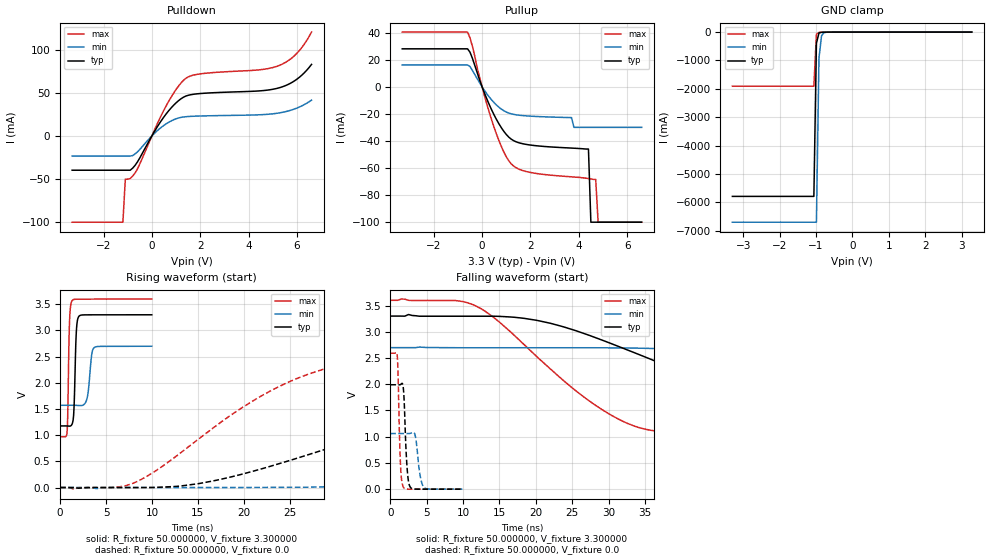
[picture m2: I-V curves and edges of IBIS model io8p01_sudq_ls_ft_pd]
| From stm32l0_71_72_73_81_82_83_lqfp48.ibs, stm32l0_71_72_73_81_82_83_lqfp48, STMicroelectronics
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|   Model io8p01_sudq_ls_ft_pd
[Model]  io8p01_sudq_ls_ft_pd
Model_type I/O
Polarity   Non-Inverting
Enable   Active-Low
Vinl =   0.990000V
Vinh =   2.310000V
Vmeas =  1.650000V
Cref =   50.000000pF
Rref =   100.000000M
Vref =   0.0V
C_comp   2.343000pF   2.309800pF   2.393900pF
[Temperature Range]   25.000000   0.125000k   -40.000000
[Pullup Reference]   3.300000V   2.700000V   3.600000V
[Pulldown Reference]   0.0V   0.0V   0.0V
[POWER Clamp Reference]   3.300000V   2.700000V   3.600000V
[GND Clamp Reference]   0.0V   0.0V   0.0V
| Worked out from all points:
|   slope of the pulldown table from 0 to 0.495 V, typ, clamps not added: 22.6 ohm
|   slope of the pullup table from 0 to 0.495 V, typ, clamps not added: 23.9 ohm
|   GND clamp passes 1 mA (typ) near -0.64 V on its own axis
|   rising waveform, R_fixture 50.000000, V_fixture 3.300000: 20-80 % time 207ps typ, 362ps min, 164ps max; typ from 1.18 V to 3.3 V
|   rising waveform, R_fixture 50.000000, V_fixture 0.0: 20-80 % time 27.1ns typ, 59.7ns min, 13.6ns max; typ from 0 V to 1.99 V
|   falling waveform, R_fixture 50.000000, V_fixture 3.300000: 20-80 % time 24.5ns typ, 54ns min, 13.4ns max; typ from 3.3 V to 1.18 V
|   falling waveform, R_fixture 50.000000, V_fixture 0.0: 20-80 % time 380ps typ, 551ps min, 301ps max; typ from 1.99 V to 0 V
[Pulldown]
|Voltage   I(typ)   I(min)   I(max)
-3.3V     -39.8mA    -23.38mA   -100mA
-1.2V     -39.8mA    -23.38mA   -100mA
-1.1V     -39.8mA    -23.38mA   -50.11mA
-900mV    -39.8mA    -23.38mA   -49.43mA
-700mV    -34.25mA   -21mA      -43.13mA
600mV     25.84mA    14.18mA    35.34mA
1V        38.32mA    19.82mA    53.81mA
1.4V      46.09mA    22.19mA    66.63mA
2V        49.05mA    23.02mA    71.83mA
5.2V      55.23mA    26.32mA    80.92mA
6V        65.76mA    32.26mA    95.84mA
6.6V      82.81mA    41.44mA    120.2mA
[Pullup]
|Voltage   I(typ)   I(min)   I(max)
-3.3V     27.97mA    16.07mA    40.33mA
-600mV    27.97mA    16.07mA    40.33mA
400mV     -17.21mA   -9.813mA   -24.69mA
800mV     -30.32mA   -16.54mA   -44.19mA
1.2V      -38.62mA   -19.99mA   -56.79mA
3.7V      -45.29mA   -22.8mA    -66.51mA
3.8V      -45.39mA   -30mA      -66.64mA
4.4V      -46mA      -30mA      -67.77mA
4.5V      -100mA     -30mA      -68.06mA
4.7V      -100mA     -30mA      -68.41mA
4.8V      -100mA     -30mA      -100mA
6.6V      -100mA     -30mA      -100mA
[GND_clamp]
|Voltage   I(typ)   I(min)   I(max)
-3.3V     -5.787A    -6.696A    -1.906A
-1.06V    -5.787A    -6.696A    -1.906A
-990mV    -393.4mA   -6.696A    -70.76mA
-920mV    -33.04mA   -919.4mA   -10.91mA
-850mV    -6.842mA   -131.3mA   -6.529mA
-780mV    -3.49mA    -21.08mA   -4.216mA
3.28V     73.94uA    88.61uA    51.47uA
[POWER_clamp]
|Voltage   I(typ)   I(min)   I(max)
-3.28V    0A         0A         0A
0V        0A         0A         0A
[Ramp]
| variable   typ   min   max
dV/dt_r  1.19406/27.10655n   0.63462/59.72155n   1.55520/13.62003n
dV/dt_f  1.27368/24.43050n   0.67098/53.94500n   1.57766/13.41415n
R_load = 50.000000
[Rising Waveform]
R_fixture= 50.000000
V_fixture= 3.300000
V_fixture_min= 2.700000
V_fixture_max= 3.600000
|time   V(typ)   V(min)   V(max)
0s        1.176V     1.571V     970mV
760.8ps   1.175V     1.571V     1.077V
1.021ns   1.172V     1.571V     3.169V
1.301ns   1.212V     1.571V     3.57V
1.502ns   1.495V     1.571V     3.592V
1.782ns   3.031V     1.569V     3.597V
2.042ns   3.27V      1.566V     3.597V
2.923ns   3.298V     1.699V     3.598V
3.744ns   3.298V     2.678V     3.598V
9.97ns    3.299V     2.698V     3.599V
[Rising Waveform]
R_fixture= 50.000000
V_fixture= 0.0
V_fixture_min= 0.0
V_fixture_max= 0.0
|time   V(typ)   V(min)   V(max)
0s        -353.6nV   -2.198uV   -103.3nV
8.008ns   -454.4uV   -168.6uV   85.67mV
15.02ns   72.49mV    -163.9uV   918.6mV
24.52ns   491.6mV    3.625mV    1.986V
30.03ns   793.5mV    19.42mV    2.322V
38.04ns   1.187V     64.52mV    2.509V
57.06ns   1.742V     269.9mV    2.583V
80.08ns   1.938V     564.8mV    2.591V
138.1ns   1.989V     964.2mV    2.592V
249.2ns   1.99V      1.06V      2.592V
[Falling Waveform]
R_fixture= 50.000000
V_fixture= 3.300000
V_fixture_min= 2.700000
V_fixture_max= 3.600000
|time   V(typ)   V(min)   V(max)
0s        3.299V     2.698V     3.599V
11.51ns   3.296V     2.695V     3.509V
20.02ns   3.221V     2.695V     2.542V
29.03ns   2.845V     2.695V     1.524V
33.53ns   2.602V     2.689V     1.203V
39.04ns   2.293V     2.669V     1.065V
56.56ns   1.482V     2.521V     988.3mV
76.58ns   1.263V     2.249V     974.4mV
131.1ns   1.184V     1.709V     970.1mV
249.2ns   1.176V     1.571V     970mV
[Falling Waveform]
R_fixture= 50.000000
V_fixture= 0.0
V_fixture_min= 0.0
V_fixture_max= 0.0
|time   V(typ)   V(min)   V(max)
0s        1.99V      1.06V      2.592V
961ps     1.99V      1.06V      2.538V
1.401ns   1.995V     1.06V      479mV
1.782ns   1.939V     1.06V      42.69mV
2.302ns   422.6mV    1.06V      1.577mV
2.763ns   36.41mV    1.064V     -28.01uV
3.423ns   857.9uV    1.022V     -51.44uV
4.104ns   1.167uV    259.3mV    -48.7uV
4.665ns   -7.715uV   27.71mV    -44.69uV
9.97ns    -353.6nV   -2.198uV   -103.3nV
